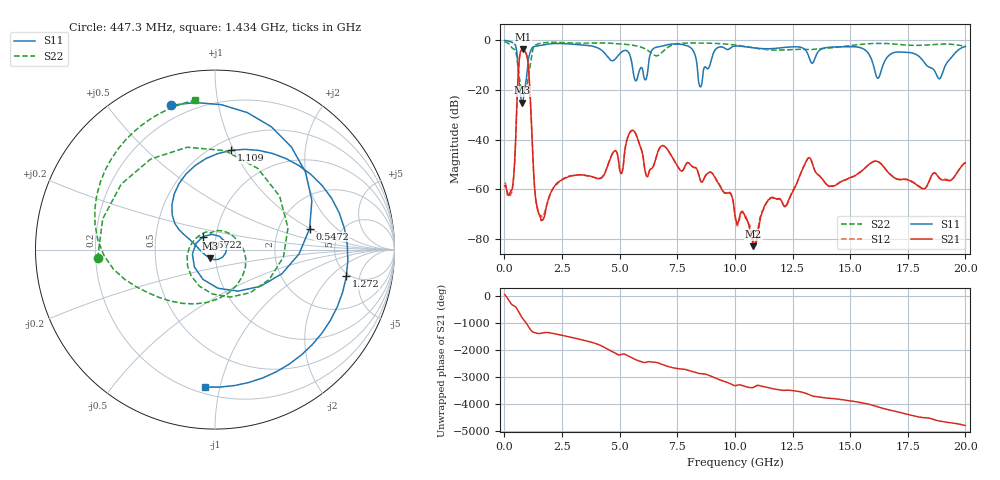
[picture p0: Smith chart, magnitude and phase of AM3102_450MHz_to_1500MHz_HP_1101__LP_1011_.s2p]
!Agilent Technologies,E8364B,MY43040894,A.07.50.67
!Agilent E8364B: A.07.50.67
!Date: Thursday, January 11, 2018 06:40:07
!Correction: S11(Full 2 Port(1,2))
!S21(Full 2 Port(1,2))
!S12(Full 2 Port(1,2))
!S22(Full 2 Port(1,2))
!S2P File: Measurements: S11, S21, S12, S22:
# Hz S  dB  R 50
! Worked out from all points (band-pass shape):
!   1601 points, 10 MHz to 20 GHz, reference 50 ohm
!   highest |S21| = -3.69 dB at 797.1 MHz (marker M1); lowest = -82.9 dB at 10.8 GHz (marker M2)
!   |S21| within 3 dB of the highest: 660 MHz to 984.5 MHz (324.5 MHz wide, 39.5 % of centre)
!   lowest |S11| = -25.1 dB at 784.6 MHz (marker M3), VSWR 1.12, Z = 47.2 - j4.59 ohm
!   |S11| at or under -10 dB: 5.544 GHz to 6.247 GHz (702.7 MHz wide, 11.9 % of centre); 8.358 GHz to 8.916 GHz (557.5 MHz wide, 6.45 % of centre); 18.31 GHz to 19.14 GHz (828.8 MHz wide, 4.43 % of centre)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
!   |S22| runs from -20.6 to -0.5 dB; largest |S21 - S12| = 0.001
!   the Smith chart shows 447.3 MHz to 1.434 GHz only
!   S11 on the Smith chart (normalised r, x): 447.3 MHz: 0.13, +0.73; 547.2 MHz: 2.99, +0.98; 672.2 MHz: 0.87, +0.13; 1.109 GHz: 0.60, +0.97; 1.272 GHz: 4.70, -3.16; 1.434 GHz: 0.24, -0.90
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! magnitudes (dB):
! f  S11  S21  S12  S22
! 10 MHz  -0.1  -58.6  -57.3  -0.5
! 272.4 MHz  -0.6  -60.6  -62.2  -2.3
! 447.3 MHz  -1.5  -48.6  -49.2  -3.7
! 547.2 MHz  -5.4  -24.5  -24.6  -7.4
! 672.2 MHz  -20.2  -5.9  -5.9  -16.8
! 784.6 MHz  -25.1  -3.7  -3.7  -19.8
! 797.1 MHz  -24.9  -3.7  -3.7  -20.2
! 1.109 GHz  -5.0  -20.5  -20.5  -10.5
! 1.272 GHz  -2.5  -53.8  -53.9  -2.8
! 1.434 GHz  -2.3  -68.0  -67.6  -1.5
! 3.346 GHz  -1.9  -54.1  -54.2  -1.1
! 5.707 GHz  -16.3  -37.8  -37.8  -2.2
! 6.182 GHz  -14.6  -54.9  -54.5  -3.8
! 6.682 GHz  -2.7  -44.3  -44.4  -6.0
! 8.081 GHz  -3.0  -50.2  -50.2  -1.1
! 8.506 GHz  -18.7  -56.4  -56.3  -1.1
! 10.01 GHz  -2.3  -70.4  -70.5  -1.9
! 10.8 GHz  -3.0  -82.9  -81.0  -3.0
! 13.34 GHz  -9.2  -49.0  -49.0  -3.7
! 16.68 GHz  -6.1  -53.4  -53.5  -1.3
! 18.86 GHz  -15.5  -55.4  -55.4  -1.5
! 20 GHz  -2.5  -49.4  -49.2  -2.3
